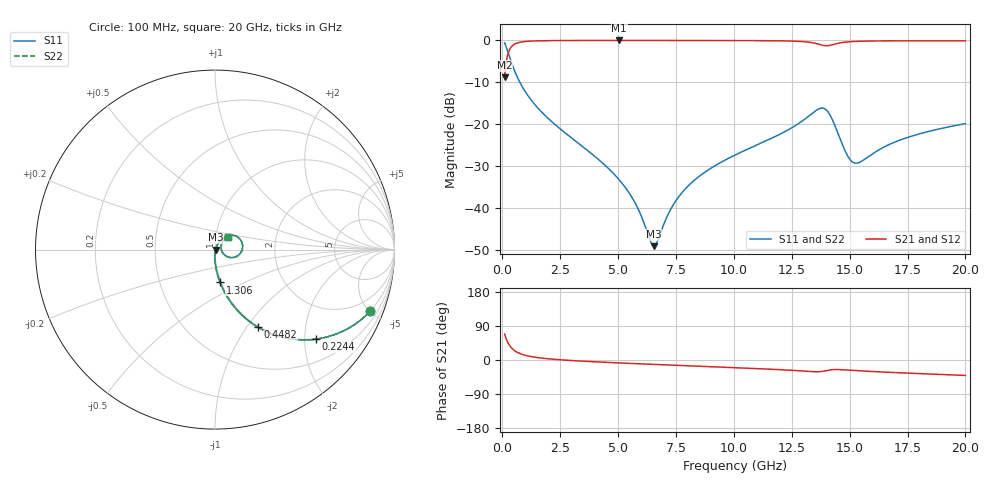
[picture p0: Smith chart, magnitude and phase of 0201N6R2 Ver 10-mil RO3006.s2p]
# GHz S MA R 50
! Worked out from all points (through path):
!   1601 points, 100 MHz to 20 GHz, reference 50 ohm
!   highest |S21| = -0.03 dB at 5.05 GHz (marker M1); lowest = -8.8 dB at 100 MHz (marker M2)
!   group delay of S21, straight-line fit = 7.41 ps
!   lowest |S11| = -49.1 dB at 6.543 GHz (marker M3), VSWR 1.01, Z = 50.3 - j0.0867 ohm
!   |S11| at or under -10 dB: 757.5 MHz to end of sweep
!   |S22| runs from -49.1 to -0.6 dB; largest |S21 - S12| = 0
!   S11 on the Smith chart (normalised r, x): 100 MHz: 0.99, -5.08; 224.4 MHz: 0.99, -2.26; 448.2 MHz: 0.99, -1.13; 1.306 GHz: 0.99, -0.37; 20 GHz: 1.14, +0.16
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0.1  0.9312 -21.5  0.3639 68.5  0.3639 68.5  0.9312 -21.5
0.224375  0.7512 -41.6  0.6592 48.3  0.6592 48.3  0.7512 -41.6
0.44825  0.4938 -61.1  0.8685 28.8  0.8685 28.8  0.4938 -61.1
0.7591875  0.3156 -72.7  0.9477 17.0  0.9477 17.0  0.3156 -72.7
1.306437  0.1851 -81.2  0.9812 8.3  0.9812 8.3  0.1851 -81.2
3.420812  0.05532 -90.4  0.9959 -2.9  0.9959 -2.9  0.05532 -90.4
5.050125  0.02163 -89.8  0.9966 -7.8  0.9966 -7.8  0.02163 -89.8
5.746625  0.01133 -83.0  0.9966 -9.6  0.9966 -9.6  0.01133 -83.0
6.542625  0.003498 -14.3  0.9963 -11.6  0.9963 -11.6  0.003498 -14.3
6.741625  0.004273 21.4  0.9963 -12.1  0.9963 -12.1  0.004273 21.4
7.264  0.009547 53.5  0.996 -13.4  0.996 -13.4  0.009547 53.5
7.885875  0.01667 61.3  0.9957 -15.0  0.9957 -15.0  0.01667 61.3
8.781375  0.02708 63.6  0.995 -17.1  0.995 -17.1  0.02708 63.6
10.05  0.04276 62.7  0.9936 -20.3  0.9936 -20.3  0.04276 62.7
12.25144  0.08266 54.9  0.9838 -26.4  0.9838 -26.4  0.08266 54.9
13.37081  0.1336 35.9  0.939 -30.6  0.939 -30.6  0.1336 35.9
13.75638  0.1551 14.9  0.8849 -30.6  0.8849 -30.6  0.1551 14.9
14.03  0.1443 -7.1  0.8632 -27.6  0.8632 -27.6  0.1443 -7.1
14.87575  0.04375 -20.5  0.9561 -26.5  0.9561 -26.5  0.04375 -20.5
15.18669  0.03459 1.7  0.9693 -27.7  0.9693 -27.7  0.03459 1.7
16.69162  0.05682 44.8  0.9856 -32.5  0.9856 -32.5  0.05682 44.8
20  0.1015 44.6  0.986 -40.7  0.986 -40.7  0.1015 44.6
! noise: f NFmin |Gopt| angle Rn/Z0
0.1  0.0007575  0.9433  0.4299  0.002989
2.301  0.004271  0.7862  4.273  0.004102
4.515  0.007111  0.7531  8.124  0.005785
6.729  0.009723  0.7344  11.97  0.007233
8.943  0.01255  0.7284  15.8  0.009025
11.14  0.01745  0.754  19.6  0.01392
13.36  0.05302  0.8956  23.54  0.1062
15.57  0.03611  0.8286  27.37  0.04189
17.79  0.02615  0.7437  30.99  0.01906
20  0.02553  0.7121  34.57  0.01598
